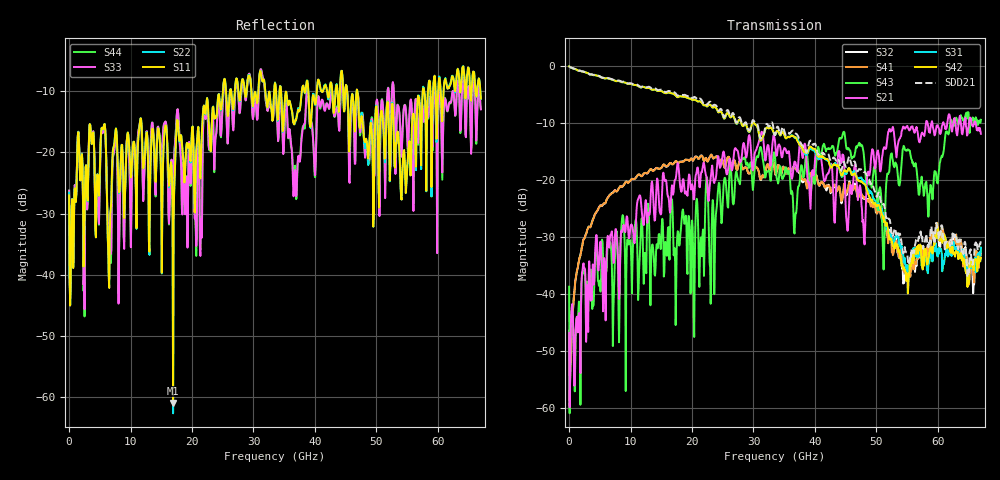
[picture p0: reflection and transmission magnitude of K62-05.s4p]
!Agilent Technologies,N5247A,US50470101,A.10.25.02
!Agilent N5247A: A.10.25.02
!Date: Tuesday, May 12, 2015 13:38:49
!Correction: Sdd11(Full 4 Port(1,2,3,4))
!Sdc11(Full 4 Port(1,2,3,4))
!Sdd12(Full 4 Port(1,2,3,4))
!Sdc12(Full 4 Port(1,2,3,4))
!Scd11(Full 4 Port(1,2,3,4))
!Scc11(Full 4 Port(1,2,3,4))
!Scd12(Full 4 Port(1,2,3,4))
!Scc12(Full 4 Port(1,2,3,4))
!Sdd21(Full 4 Port(1,2,3,4))
!Sdc21(Full 4 Port(1,2,3,4))
!Sdd22(Full 4 Port(1,2,3,4))
!Sdc22(Full 4 Port(1,2,3,4))
!Scd21(Full 4 Port(1,2,3,4))
!Scc21(Full 4 Port(1,2,3,4))
!Scd22(Full 4 Port(1,2,3,4))
!Scc22(Full 4 Port(1,2,3,4))
!Balanced Topology: BBAL
!S4P File: Measurements: <Sdd11,Sdc11,Sdd12,Sdc12>,
!<Scd11,Scc11,Scd12,Scc12>,
!<Sdd21,Sdc21,Sdd22,Sdc22>,
!<Scd21,Scc21,Scd22,Scc22>:
# Hz S  dB  R 50
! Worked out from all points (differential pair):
!   801 points, 10 MHz to 67 GHz, reference 50 ohm
!   strongest paths, dB at 10 MHz, 16.76 GHz, 33.51 GHz, 50.25 GHz, 67 GHz:
!     S42: 0.0, -4.8, -12.1, -24.4, -33.7
!     S31: 0.0, -4.8, -12.1, -24.5, -31.8
!     S21: -46.9, -20.9, -13.2, -14.8, -11.9
!     S43: -38.7, -23.4, -15.9, -25.3, -9.4
!     S41: -59.4, -17.2, -18.7, -25.5, -33.0
!     S32: -46.4, -17.2, -18.7, -25.2, -32.9
!   taken as a pair (ports 2,1 in; 4,3 out), SDD21 dB: 0.0, -4.5, -12.1, -22.4, -30.5
!   lowest |S11| = -60.9 dB at 16.92 GHz (marker M1), VSWR 1.00, Z = 49.9 - j0.0516 ohm
!   |S11| at or under -10 dB: start of sweep to 25.04 GHz; 34.48 GHz to 37.88 GHz (3.398 GHz wide, 9.39 % of centre); 46.9 GHz to 57.55 GHz (10.65 GHz wide, 20.4 % of centre)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
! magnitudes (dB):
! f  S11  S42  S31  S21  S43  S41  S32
! 10 MHz  -27.0  0.0  0.0  -46.9  -38.7  -59.4  -46.4
! 2.941 GHz  -27.1  -1.2  -1.2  -38.5  -37.8  -28.7  -28.8
! 16.92 GHz  -60.9  -4.8  -4.8  -22.6  -28.5  -17.2  -17.2
! 25.3 GHz  -8.0  -9.2  -9.2  -15.9  -19.6  -17.8  -17.8
! 44.56 GHz  -9.1  -18.8  -19.3  -15.5  -11.8  -22.4  -22.5
! 51.17 GHz  -16.9  -26.4  -26.7  -14.5  -35.7  -27.2  -26.9
! 67 GHz  -11.2  -33.7  -31.8  -11.9  -9.4  -33.0  -32.9
